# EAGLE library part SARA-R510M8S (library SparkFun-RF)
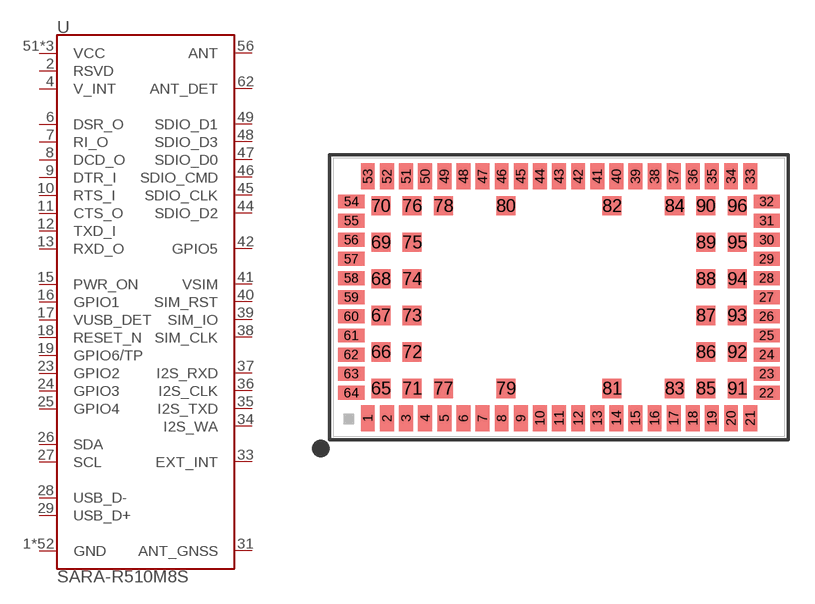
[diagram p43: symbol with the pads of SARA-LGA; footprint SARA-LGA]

Designator prefix U

## SARA-R510M8S (PROD_ID: IC-15573; VALUE: SARA-R510M8S)  [SARA-LGA]
1  GND  pwr
2  RSVD  nc
3  GND  pwr
4  V_INT  out
5  GND  pwr
6  DSR_O  out
7  RI_O  out
8  DCD_O  out
9  DTR_I  in
10  RTS_I  in
11  CTS_O  out
12  TXD_I  in
13  RXD_O  out
14  GND  pwr
15  PWR_ON  in
16  GPIO1
17  VUSB_DET  in
18  RESET_N  in
19  GPIO6/TP
20  GND  pwr
21  GND  pwr
22  GND  pwr
23  GPIO2
24  GPIO3
25  GPIO4
26  SDA
27  SCL
28  USB_D-
29  USB_D+
30  GND  pwr
31  ANT_GNSS  in
32  GND  pwr
33  EXT_INT  in
34  I2S_WA  out
35  I2S_TXD  out
36  I2S_CLK  out
37  I2S_RXD  in
38  SIM_CLK  out
39  SIM_IO
40  SIM_RST  out
41  VSIM  out
42  GPIO5
43  GND  pwr
44  SDIO_D2
45  SDIO_CLK  out
46  SDIO_CMD
47  SDIO_D0
48  SDIO_D3
49  SDIO_D1
50  GND  pwr
51  VCC  pwr
52  VCC  pwr
53  VCC  pwr
54  GND  pwr
55  GND  pwr
56  ANT
57  GND  pwr
58  GND  pwr
59  GND  pwr
60  GND  pwr
61  GND  pwr
62  ANT_DET  in
63  GND  pwr
64  GND  pwr
65  GND  pwr
66  GND  pwr
67  GND  pwr
68  GND  pwr
69  GND  pwr
70  GND  pwr
71  GND  pwr
72  GND  pwr
73  GND  pwr
74  GND  pwr
75  GND  pwr
76  GND  pwr
77  GND  pwr
78  GND  pwr
79  GND  pwr
80  GND  pwr
81  GND  pwr
82  GND  pwr
83  GND  pwr
84  GND  pwr
85  GND  pwr
86  GND  pwr
87  GND  pwr
88  GND  pwr
89  GND  pwr
90  GND  pwr
91  GND  pwr
92  GND  pwr
93  GND  pwr
94  GND  pwr
95  GND  pwr
96  GND  pwr

## Footprint SARA-LGA (pad centres in mm)
ublox SARA LGA form factor Miniature cellular modem package. Common form factor for many ublox cellular modules, including SARA-R4 and SARA-U2 series. Dimensions: 26.0 x 16.0 mm Pins: 96 Pitch: 1.1mm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
smd 0.8 x 1.5: 1 -11,-6.95; 2 -9.9,-6.95; 3 -8.8,-6.95; 4 -7.7,-6.95; 5 -6.6,-6.95; 6 -5.5,-6.95; 7 -4.4,-6.95; 8 -3.3,-6.95; 9 -2.2,-6.95; 10 -1.1,-6.95; 11 0,-6.95; 12 1.1,-6.95; 13 2.2,-6.95; 14 3.3,-6.95; 15 4.4,-6.95; 16 5.5,-6.95; 17 6.6,-6.95; 18 7.7,-6.95; 19 8.8,-6.95; 20 9.9,-6.95; 21 11,-6.95; 33 11,6.95; 34 9.9,6.95; 35 8.8,6.95; 36 7.7,6.95; 37 6.6,6.95; 38 5.5,6.95; 39 4.4,6.95; 40 3.3,6.95; 41 2.2,6.95; 42 1.1,6.95; 43 0,6.95; 44 -1.1,6.95; 45 -2.2,6.95; 46 -3.3,6.95; 47 -4.4,6.95; 48 -5.5,6.95; 49 -6.6,6.95; 50 -7.7,6.95; 51 -8.8,6.95; 52 -9.9,6.95; 53 -11,6.95
smd 1.5 x 0.8: 22 11.95,-5.5; 23 11.95,-4.4; 24 11.95,-3.3; 25 11.95,-2.2; 26 11.95,-1.1; 27 11.95,0; 28 11.95,1.1; 29 11.95,2.2; 30 11.95,3.3; 31 11.95,4.4; 32 11.95,5.5; 54 -11.95,5.5; 55 -11.95,4.4; 56 -11.95,3.3; 57 -11.95,2.2; 58 -11.95,1.1; 59 -11.95,0; 60 -11.95,-1.1; 61 -11.95,-2.2; 62 -11.95,-3.3; 63 -11.95,-4.4; 64 -11.95,-5.5
smd 1.1 x 1.1: 65 -10.25,-5.25; 66 -10.25,-3.15; 67 -10.25,-1.05; 68 -10.25,1.05; 69 -10.25,3.15; 70 -10.25,5.25; 71 -8.45,-5.25; 72 -8.45,-3.15; 73 -8.45,-1.05; 74 -8.45,1.05; 75 -8.45,3.15; 76 -8.45,5.25; 77 -6.65,-5.25; 78 -6.65,5.25; 79 -3.05,-5.25; 80 -3.05,5.25; 81 3.05,-5.25; 82 3.05,5.25; 83 6.65,-5.25; 84 6.65,5.25; 85 8.45,-5.25; 86 8.45,-3.15; 87 8.45,-1.05; 88 8.45,1.05; 89 8.45,3.15; 90 8.45,5.25; 91 10.25,-5.25; 92 10.25,-3.15; 93 10.25,-1.05; 94 10.25,1.05; 95 10.25,3.15; 96 10.25,5.25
